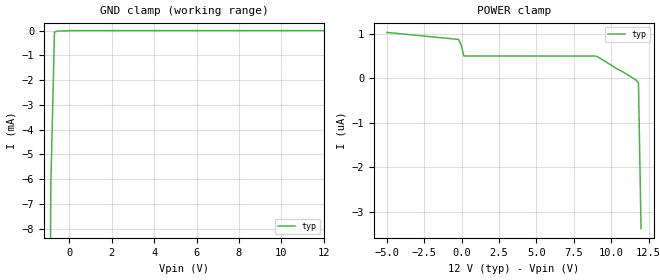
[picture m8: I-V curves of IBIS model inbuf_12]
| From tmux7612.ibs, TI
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| inbuf_12
[Model]   inbuf_12
Model_type   Input
Vinl = 0.8
Vinh = 1.3
|   typ   min   max
C_comp   1.598234e-12   NA   NA
[Voltage Range]   12   NA   NA
[Temperature Range]   27   NA   NA
[Power Clamp Reference]   12   NA   NA
[GND Clamp Reference]   0   NA   NA
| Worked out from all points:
|   GND clamp passes 1 mA (typ) near -0.73 V on its own axis
[GND Clamp]
|   Voltage   I(typ)   I(min)   I(max)
-5V       -3.924A    NA         NA
-1.051V   -33.79mA   NA         NA
-878.8mV  -6.21mA    NA         NA
-707.1mV  -61.9uA    NA         NA
-535.4mV  -13.46uA   NA         NA
151.5mV   -136.7nA   NA         NA
12V       680.7nA    NA         NA
[POWER Clamp]
|   Voltage   I(typ)   I(min)   I(max)
-5V       1.031uA    NA         NA
-191.9mV  871.7nA    NA         NA
-20.2mV   744.3nA    NA         NA
151.5mV   501.5nA    NA         NA
8.909V    499.2nA    NA         NA
9.081V    484.8nA    NA         NA
11.66V    -39.31nA   NA         NA
11.83V    -102.7nA   NA         NA
12V       -3.385uA   NA         NA
